[IBIS Ver]   5.1
[File name]   imx8mn_v1.ibs
[File Rev]   1.0
[Date]   Apr 12,2021
[Notes]   One-Section RLC
[Component] imx8mn_14x14_v1
[Manufacturer] Manufacturer_Name
[Package]
|   typ   min   max
R_pkg   0.39844   0.18702   0.658
L_pkg   2.971e-9   1.249e-9   5.232e-9
C_pkg   8.434e-13   5.175e-13   1.203e-12
[Pin]   Signal_name   model_name   R_pin   L_pin   C_pin
M19 NVCC_CLK POWER
K8 NVCC_DRAM POWER
K9 NVCC_DRAM POWER
L9 NVCC_DRAM POWER
M9 NVCC_DRAM POWER
N8 NVCC_DRAM POWER
N9 NVCC_DRAM POWER
P7 NVCC_DRAM POWER
R8 NVCC_DRAM POWER
R9 NVCC_DRAM POWER
T9 NVCC_DRAM POWER
U9 NVCC_DRAM POWER
V8 NVCC_DRAM POWER
V9 NVCC_DRAM POWER
H10 NVCC_ECSPI POWER
W22 NVCC_ENET POWER
W12 NVCC_GPIO1 POWER
J11 NVCC_I2C POWER
L19 NVCC_JTAG POWER
U19 NVCC_NAND POWER
V19 NVCC_SAI2 POWER
Y10 NVCC_SAI3 POWER
W17 NVCC_SAI5 POWER
V20 NVCC_SD1 POWER
V22 NVCC_SD2 POWER
J22 NVCC_SNVS_1P8 POWER
J12 NVCC_UART POWER
AB13 PVCC0_1P8 POWER
T19 PVCC1_1P8 POWER
J13 PVCC2_1P8 POWER
N19 VDD_24M_XTAL_1P8 POWER
AA14 VDD_ANA0_1P8 POWER
Y15 VDD_ANA0_1P8 POWER
N20 VDD_ANA1_1P8 POWER
P19 VDD_ANA1_1P8 POWER
L17 VDD_ANA_0P8 POWER
N17 VDD_ANA_0P8 POWER
R13 VDD_ARM POWER
R15 VDD_ARM POWER
T13 VDD_ARM POWER
T14 VDD_ARM POWER
T15 VDD_ARM POWER
U13 VDD_ARM POWER
U15 VDD_ARM POWER
V13 VDD_ARM POWER
V15 VDD_ARM POWER
V16 VDD_ARM POWER
W13 VDD_ARM POWER
W14 VDD_ARM POWER
W15 VDD_ARM POWER
W16 VDD_ARM POWER
P16 VDD_ARM_PLL_0P8 POWER
R19 VDD_ARM_PLL_1P8 POWER
J10 VDD_DRAM POWER
L10 VDD_DRAM POWER
N10 VDD_DRAM POWER
R10 VDD_DRAM POWER
U10 VDD_DRAM POWER
W10 VDD_DRAM POWER
P9 VDD_DRAM_PLL_0P8 POWER
P5 VDD_DRAM_PLL_1P8 POWER
P12 VDD_GPU POWER
R11 VDD_GPU POWER
U11 VDD_GPU POWER
V12 VDD_GPU POWER
W11 VDD_GPU POWER
J14 VDD_MIPI_0P8 POWER
J15 VDD_MIPI_1P2 POWER
H13 VDD_MIPI_1P8 POWER
K22 VDD_SNVS_0P8 POWER
K15 VDD_SOC POWER
K16 VDD_SOC POWER
L15 VDD_SOC POWER
L18 VDD_SOC POWER
M15 VDD_SOC POWER
N13 VDD_SOC POWER
N15 VDD_SOC POWER
N18 VDD_SOC POWER
R17 VDD_SOC POWER
R18 VDD_SOC POWER
U17 VDD_SOC POWER
U18 VDD_SOC POWER
J17 VDD_USB_0P8 POWER
H15 VDD_USB_1P8 POWER
K19 VDD_USB_3P3 POWER
P1 DRAM_VREF POWER
B27 24M_XTALI NC 0.51574 3.88E-09 9.69E-13
C26 24M_XTALO NC 0.47173 3.65E-09 9.10E-13
G26 BOOT_MODE0 PBIDIRHS_E33_33_NT_DR_H 0.46814 3.31E-09 8.70E-13
G27 BOOT_MODE1 PBIDIRHS_E33_33_NT_DR_H 0.42497 3.31E-09 8.83E-13
C27 BOOT_MODE2 PBIDIRHS_E33_33_NT_DR_H 0.658 4.64E-09 1.10E-12
D26 BOOT_MODE3 PBIDIRHS_E33_33_NT_DR_H 0.45096 3.50E-09 9.48E-13
H27 CLKIN1 PBIDIRHS_E33_33_NT_DR_H 0.42819 3.10E-09 8.46E-13
J27 CLKIN2 PBIDIRHS_E33_33_NT_DR_H 0.39512 2.88E-09 8.19E-13
H26 CLKOUT1 PBIDIRHS_E33_33_NT_DR_H 0.42258 3.09E-09 8.72E-13
J26 CLKOUT2 PBIDIRHS_E33_33_NT_DR_H 0.38896 2.86E-09 8.59E-13
F4 DRAM_AC00 CA_CK 0.48824 3.22E-09 9.34E-13
F5 DRAM_AC01 CA_CK 0.35707 2.39E-09 8.27E-13
K4 DRAM_AC02 CA_CK 0.39984 2.51E-09 6.33E-13
J4 DRAM_AC03 CA_CK 0.4301 2.77E-09 8.38E-13
L2 DRAM_AC04 CA_CK 0.36588 2.48E-09 7.90E-13
L1 DRAM_AC05 CA_CK 0.36576 2.54E-09 7.85E-13
F6 DRAM_AC06 CA_CK 0.4007 2.77E-09 8.84E-13
J5 DRAM_AC07 CA_CK 0.32797 2.10E-09 7.49E-13
J6 DRAM_AC08 CA_CK 0.37592 2.45E-09 7.51E-13
K6 DRAM_AC09 CA_CK 0.2687 1.75E-09 6.37E-13
E4 DRAM_AC10 CA_CK 0.47313 3.25E-09 1.07E-12
D5 DRAM_AC11 CA_CK 0.5424 3.66E-09 1.09E-12
N4 DRAM_AC12 CA_CK 0.31375 2.03E-09 7.30E-13
N5 DRAM_AC13 CA_CK 0.3154 2.11E-09 5.26E-13
K5 DRAM_AC14 CA_CK 0.38927 2.66E-09 8.12E-13
N6 DRAM_AC15 CA_CK 0.19955 1.25E-09 5.44E-13
M1 DRAM_AC16 CA_CK 0.35347 2.44E-09 7.55E-13
M2 DRAM_AC17 CA_CK 0.358 2.43E-09 7.51E-13
N2 DRAM_AC19 CA_CK 0.40801 2.75E-09 7.90E-13
AB4 DRAM_AC20 CA_CK 0.42345 3.02E-09 1.01E-12
AB5 DRAM_AC21 CA_CK 0.42752 3.07E-09 9.99E-13
W4 DRAM_AC22 CA_CK 0.4158 2.93E-09 8.70E-13
V4 DRAM_AC23 CA_CK 0.32528 2.28E-09 8.23E-13
U2 DRAM_AC24 CA_CK 0.39035 2.60E-09 7.87E-13
U1 DRAM_AC25 CA_CK 0.38541 2.61E-09 8.04E-13
N1 DRAM_AC26 CA_CK 0.44985 3.23E-09 9.76E-13
R6 DRAM_AC27 CA_CK 0.25296 1.74E-09 5.79E-13
W6 DRAM_AC28 CA_CK 0.24654 1.73E-09 6.92E-13
V6 DRAM_AC29 CA_CK 0.2963 2.07E-09 6.79E-13
AC4 DRAM_AC30 CA_CK 0.49352 3.59E-09 1.07E-12
AD5 DRAM_AC31 CA_CK 0.4395 3.25E-09 1.10E-12
R4 DRAM_AC32 CA_CK 0.27402 1.95E-09 7.28E-13
R5 DRAM_AC33 CA_CK 0.33648 2.47E-09 7.04E-13
T1 DRAM_AC34 CA_CK 0.33909 2.47E-09 8.79E-13
T2 DRAM_AC35 CA_CK 0.4206 3.03E-09 9.57E-13
V5 DRAM_AC36 CA_CK 0.21143 1.53E-09 5.18E-13
W5 DRAM_AC37 CA_CK 0.27343 2.01E-09 7.34E-13
AB6 DRAM_AC38 CA_CK 0.3378 2.47E-09 7.95E-13
R2 DRAM_ALERT_N CA_CK 0.32975 2.21E-09 7.44E-13
A4 DRAM_DM0 DQ_DQS 0.49985 3.46E-09 1.04E-12
F1 DRAM_DM1 DQ_DQS 0.5397 3.63E-09 1.05E-12
A5 DRAM_DQ00 DQ_DQS 0.39147 2.99E-09 8.20E-13
B5 DRAM_DQ01 DQ_DQS 0.3615 2.50E-09 8.23E-13
D2 DRAM_DQ02 DQ_DQS 0.47251 3.12E-09 9.96E-13
D1 DRAM_DQ03 DQ_DQS 0.41907 2.95E-09 9.98E-13
C1 DRAM_DQ04 DQ_DQS 0.59741 3.79E-09 1.09E-12
B1 DRAM_DQ05 DQ_DQS 0.54423 3.70E-09 9.92E-13
A3 DRAM_DQ06 DQ_DQS 0.59637 3.94E-09 1.17E-12
B4 DRAM_DQ07 DQ_DQS 0.44773 2.99E-09 1.01E-12
F2 DRAM_DQ08 DQ_DQS 0.41874 2.65E-09 8.49E-13
G2 DRAM_DQ09 DQ_DQS 0.49278 3.11E-09 8.75E-13
J1 DRAM_DQ10 DQ_DQS 0.40348 2.71E-09 9.07E-13
J2 DRAM_DQ11 DQ_DQS 0.46658 2.91E-09 8.48E-13
K2 DRAM_DQ12 DQ_DQS 0.37348 2.33E-09 7.90E-13
K1 DRAM_DQ13 DQ_DQS 0.47478 3.06E-09 8.57E-13
E1 DRAM_DQ14 DQ_DQS 0.48488 3.33E-09 1.12E-12
E2 DRAM_DQ15 DQ_DQS 0.45234 3.01E-09 1.02E-12
B2 DRAM_DQS0_N DQ_DQS 0.53019 3.56E-09 1.07E-12
A2 DRAM_DQS0_P DQ_DQS 0.53145 3.58E-09 1.06E-12
H1 DRAM_DQS1_N DQ_DQS 0.40944 3.10E-09 8.31E-13
G1 DRAM_DQS1_P DQ_DQS 0.40431 3.20E-09 8.34E-13
R1 DRAM_RESET_N CA_CK 0.3454 2.35E-09 7.49E-13
P2 DRAM_ZN CA_CK 0.23974 1.79E-09 7.30E-13
A7 ECSPI1_MISO PBIDIRHS_E33_33_NT_DR_V 0.37355 2.89E-09 7.69E-13
B7 ECSPI1_MOSI PBIDIRHS_E33_33_NT_DR_V 0.33402 2.36E-09 7.74E-13
D6 ECSPI1_SCLK PBIDIRHS_E33_33_NT_DR_V 0.29824 2.14E-09 8.07E-13
B6 ECSPI1_SS0 PBIDIRHS_E33_33_NT_DR_V 0.33367 2.42E-09 8.63E-13
A8 ECSPI2_MISO PBIDIRHS_E33_33_NT_DR_V 0.351 2.53E-09 8.75E-13
B8 ECSPI2_MOSI PBIDIRHS_E33_33_NT_DR_V 0.34979 2.52E-09 8.27E-13
E6 ECSPI2_SCLK PBIDIRHS_E33_33_NT_DR_V 0.24339 1.77E-09 7.01E-13
A6 ECSPI2_SS0 PBIDIRHS_E33_33_NT_DR_V 0.378 2.72E-09 9.37E-13
AC27 ENET_MDC PBIDIRHS_E33_33_NT_DR_V 0.49185 3.73E-09 1.02E-12
AB27 ENET_MDIO PBIDIRHS_E33_33_NT_DR_V 0.52367 3.84E-09 1.03E-12
AE27 ENET_RD0 PBIDIRHS_E33_33_NT_DR_V 0.60251 4.83E-09 1.15E-12
AD27 ENET_RD1 PBIDIRHS_E33_33_NT_DR_V 0.58514 4.47E-09 1.11E-12
AD26 ENET_RD2 PBIDIRHS_E33_33_NT_DR_V 0.54339 4.25E-09 1.02E-12
AC26 ENET_RD3 PBIDIRHS_E33_33_NT_DR_V 0.50617 4.39E-09 9.34E-13
AE26 ENET_RXC PBIDIRHS_E33_33_NT_DR_V 0.58821 4.99E-09 1.00E-12
AF27 ENET_RX_CTL PBIDIRHS_E33_33_NT_DR_V 0.6411 4.81E-09 1.17E-12
AG26 ENET_TD0 PBIDIRHS_E33_33_NT_DR_V 0.63183 5.23E-09 1.20E-12
AF26 ENET_TD1 PBIDIRHS_E33_33_NT_DR_V 0.53971 4.66E-09 1.03E-12
AG25 ENET_TD2 PBIDIRHS_E33_33_NT_DR_V 0.56983 5.01E-09 1.01E-12
AF25 ENET_TD3 PBIDIRHS_E33_33_NT_DR_V 0.53389 4.38E-09 1.04E-12
AG24 ENET_TXC PBIDIRHS_E33_33_NT_DR_V 0.60522 4.99E-09 1.09E-12
AF24 ENET_TX_CTL PBIDIRHS_E33_33_NT_DR_V 0.49602 3.94E-09 9.36E-13
AG14 GPIO1_IO00 PBIDIRHS_E33_33_NT_DR_V 0.47303 3.55E-09 1.03E-12
AF14 GPIO1_IO01 PBIDIRHS_E33_33_NT_DR_V 0.49773 3.62E-09 9.72E-13
AG13 GPIO1_IO02 PBIDIRHS_E33_33_NT_DR_V 0.42117 3.18E-09 9.11E-13
AF13 GPIO1_IO03 PBIDIRHS_E33_33_NT_DR_V 0.43028 3.16E-09 8.20E-13
AG12 GPIO1_IO04 PBIDIRHS_E33_33_NT_DR_V 0.44738 3.29E-09 9.53E-13
AF12 GPIO1_IO05 PBIDIRHS_E33_33_NT_DR_V 0.42301 3.03E-09 8.41E-13
AG11 GPIO1_IO06 PBIDIRHS_E33_33_NT_DR_V 0.38341 2.96E-09 7.42E-13
AF11 GPIO1_IO07 PBIDIRHS_E33_33_NT_DR_V 0.42212 3.04E-09 7.78E-13
AG10 GPIO1_IO08 PBIDIRHS_E33_33_NT_DR_V 0.42061 3.41E-09 7.40E-13
AF10 GPIO1_IO09 PBIDIRHS_E33_33_NT_DR_V 0.48934 3.59E-09 9.08E-13
AD10 GPIO1_IO10 PBIDIRHS_E33_33_NT_DR_V 0.32648 2.56E-09 7.47E-13
AC10 GPIO1_IO11 PBIDIRHS_E33_33_NT_DR_V 0.40226 3.02E-09 8.33E-13
AB10 GPIO1_IO12 PBIDIRHS_E33_33_NT_DR_V 0.29622 2.30E-09 6.74E-13
AD9 GPIO1_IO13 PBIDIRHS_E33_33_NT_DR_V 0.40673 3.04E-09 8.24E-13
AC9 GPIO1_IO14 PBIDIRHS_E33_33_NT_DR_V 0.34159 2.68E-09 7.60E-13
AB9 GPIO1_IO15 PBIDIRHS_E33_33_NT_DR_V 0.38348 2.87E-09 7.64E-13
E9 I2C1_SCL PBIDIRHS_E33_33_NT_DR_V 0.25158 2.14E-09 6.92E-13
F9 I2C1_SDA PBIDIRHS_E33_33_NT_DR_V 0.19616 1.61E-09 6.06E-13
D10 I2C2_SCL PBIDIRHS_E33_33_NT_DR_V 0.27825 2.30E-09 7.25E-13
D9 I2C2_SDA PBIDIRHS_E33_33_NT_DR_V 0.27493 2.22E-09 7.43E-13
E10 I2C3_SCL PBIDIRHS_E33_33_NT_DR_V 0.21555 1.65E-09 5.84E-13
F10 I2C3_SDA PBIDIRHS_E33_33_NT_DR_V 0.19827 1.70E-09 5.71E-13
D13 I2C4_SCL PBIDIRHS_E33_33_NT_DR_V 0.33107 2.61E-09 8.61E-13
E13 I2C4_SDA PBIDIRHS_E33_33_NT_DR_V 0.29585 2.52E-09 7.61E-13
D27 JTAG_MOD PBIDIRHS_E33_33_NT_DR_V 0.60254 4.45E-09 1.11E-12
F26 JTAG_TCK PBIDIRHS_E33_33_NT_DR_V 0.4046 3.09E-09 8.46E-13
E27 JTAG_TDI PBIDIRHS_E33_33_NT_DR_V 0.50933 3.80E-09 9.77E-13
E26 JTAG_TDO PBIDIRHS_E33_33_NT_DR_V 0.55324 4.11E-09 1.02E-12
F27 JTAG_TMS PBIDIRHS_E33_33_NT_DR_V 0.52515 3.82E-09 9.81E-13
A16 MIPI_CSI_CLK_N DPHY_RX 0.45964 3.21E-09 8.86E-13
B16 MIPI_CSI_CLK_P DPHY_RX 0.44956 3.14E-09 8.89E-13
A14 MIPI_CSI_D0_N DPHY_RX 0.44549 3.14E-09 8.76E-13
B14 MIPI_CSI_D0_P DPHY_RX 0.4516 3.13E-09 8.63E-13
A15 MIPI_CSI_D1_N DPHY_RX 0.45153 3.18E-09 8.87E-13
B15 MIPI_CSI_D1_P DPHY_RX 0.46295 3.20E-09 8.68E-13
A17 MIPI_CSI_D2_N DPHY_RX 0.4619 3.26E-09 8.75E-13
B17 MIPI_CSI_D2_P DPHY_RX 0.45927 3.18E-09 8.77E-13
A18 MIPI_CSI_D3_N DPHY_RX 0.45552 3.23E-09 8.74E-13
B18 MIPI_CSI_D3_P DPHY_RX 0.45125 3.18E-09 8.80E-13
A11 MIPI_DSI_CLK_N DPHY_TX 0.4522 3.02E-09 8.88E-13
B11 MIPI_DSI_CLK_P DPHY_TX 0.44443 2.98E-09 8.65E-13
A9 MIPI_DSI_D0_N DPHY_TX 0.44051 3.11E-09 8.90E-13
B9 MIPI_DSI_D0_P DPHY_TX 0.4461 3.17E-09 8.59E-13
A10 MIPI_DSI_D1_N DPHY_TX 0.44518 3.03E-09 8.77E-13
B10 MIPI_DSI_D1_P DPHY_TX 0.44943 3.06E-09 8.56E-13
A12 MIPI_DSI_D2_N DPHY_TX 0.45489 3.23E-09 8.88E-13
B12 MIPI_DSI_D2_P DPHY_TX 0.46388 3.01E-09 8.79E-13
A13 MIPI_DSI_D3_N DPHY_TX 0.44597 3.26E-09 8.85E-13
B13 MIPI_DSI_D3_P DPHY_TX 0.45687 3.24E-09 8.67E-13
D15 MIPI_VREG_CAP NC 0.33053 2.45E-09 7.14E-13
N22 NAND_ALE PBIDIRHS_E33_33_NT_DR_H 0.26209 1.92E-09 5.56E-13
N24 NAND_CE0_B PBIDIRHS_E33_33_NT_DR_H 0.3626 3.19E-09 7.69E-13
P27 NAND_CE1_B PBIDIRHS_E33_33_NT_DR_H 0.41324 3.16E-09 8.06E-13
M27 NAND_CE2_B PBIDIRHS_E33_33_NT_DR_H 0.50235 3.88E-09 8.77E-13
L27 NAND_CE3_B PBIDIRHS_E33_33_NT_DR_H 0.41619 3.33E-09 9.27E-13
K27 NAND_CLE PBIDIRHS_E33_33_NT_DR_H 0.44944 3.60E-09 9.50E-13
P23 NAND_DATA00 PBIDIRHS_E33_33_NT_DR_H 0.23195 2.34E-09 6.09E-13
K24 NAND_DATA01 PBIDIRHS_E33_33_NT_DR_H 0.30636 2.35E-09 7.32E-13
K23 NAND_DATA02 PBIDIRHS_E33_33_NT_DR_H 0.32853 2.76E-09 8.04E-13
N23 NAND_DATA03 PBIDIRHS_E33_33_NT_DR_H 0.22735 1.98E-09 5.70E-13
M26 NAND_DATA04 PBIDIRHS_E33_33_NT_DR_H 0.43592 3.78E-09 8.40E-13
L26 NAND_DATA05 PBIDIRHS_E33_33_NT_DR_H 0.40519 3.05E-09 8.29E-13
K26 NAND_DATA06 PBIDIRHS_E33_33_NT_DR_H 0.41314 3.66E-09 9.50E-13
N26 NAND_DATA07 PBIDIRHS_E33_33_NT_DR_H 0.41424 3.08E-09 8.08E-13
R22 NAND_DQS PBIDIRHS_E33_33_NT_DR_H 0.28012 2.14E-09 6.66E-13
P26 NAND_READY_B PBIDIRHS_E33_33_NT_DR_H 0.31826 2.47E-09 7.40E-13
N27 NAND_RE_B PBIDIRHS_E33_33_NT_DR_H 0.44902 3.43E-09 8.46E-13
R26 NAND_WE_B PBIDIRHS_E33_33_NT_DR_H 0.49038 3.54E-09 9.33E-13
R27 NAND_WP_B PBIDIRHS_E33_33_NT_DR_H 0.3616 2.86E-09 8.09E-13
A25 ONOFF PINC_E33_33_NT_DR_H 0.42391 3.27E-09 9.04E-13
A24 PMIC_ON_REQ PBIDIR_E33_33_NT_DR_H 0.42415 3.44E-09 7.76E-13
E24 PMIC_STBY_REQ PBIDIR_E33_33_NT_DR_H 0.43218 3.22E-09 8.78E-13
B24 POR_B PINC_E33_33_NT_DR_H 0.43987 3.79E-09 9.00E-13
F24 RTC_RESET_B PINC_E33_33_NT_DR_H 0.29095 2.49E-09 7.04E-13
A26 RTC_XTALI NC 0.50843 4.03E-09 9.60E-13
B25 RTC_XTALO NC 0.48113 3.81E-09 9.71E-13
AD19 SAI2_MCLK PBIDIRHS_E33_33_NT_DR_V 0.34257 2.69E-09 7.35E-13
AB22 SAI2_RXC PBIDIRHS_E33_33_NT_DR_V 0.47663 3.51E-09 8.91E-13
AC24 SAI2_RXD0 PBIDIRHS_E33_33_NT_DR_V 0.56459 4.37E-09 1.02E-12
AC19 SAI2_RXFS PBIDIRHS_E33_33_NT_DR_V 0.30707 2.36E-09 6.89E-13
AD22 SAI2_TXC PBIDIRHS_E33_33_NT_DR_V 0.46249 3.50E-09 9.07E-13
AC22 SAI2_TXD0 PBIDIRHS_E33_33_NT_DR_V 0.48787 3.55E-09 9.44E-13
AD23 SAI2_TXFS PBIDIRHS_E33_33_NT_DR_V 0.56772 4.24E-09 1.04E-12
AD6 SAI3_MCLK PBIDIRHS_E33_33_NT_DR_V 0.33969 2.39E-09 7.88E-13
AG7 SAI3_RXC PBIDIRHS_E33_33_NT_DR_V 0.37044 2.73E-09 8.81E-13
AF7 SAI3_RXD PBIDIRHS_E33_33_NT_DR_V 0.36591 2.65E-09 8.38E-13
AG8 SAI3_RXFS PBIDIRHS_E33_33_NT_DR_V 0.36577 2.56E-09 8.68E-13
AG6 SAI3_TXC PBIDIRHS_E33_33_NT_DR_V 0.39305 2.73E-09 9.47E-13
AF6 SAI3_TXD PBIDIRHS_E33_33_NT_DR_V 0.35362 2.42E-09 8.58E-13
AC6 SAI3_TXFS PBIDIRHS_E33_33_NT_DR_V 0.34927 2.54E-09 8.07E-13
AD15 SAI5_MCLK PBIDIRHS_E33_33_NT_DR_V 0.29891 2.34E-09 7.29E-13
AC15 SAI5_RXC PBIDIRHS_E33_33_NT_DR_V 0.32942 2.52E-09 6.46E-13
AD18 SAI5_RXD0 PBIDIRHS_E33_33_NT_DR_V 0.33327 2.69E-09 7.85E-13
AC14 SAI5_RXD1 PBIDIRHS_E33_33_NT_DR_V 0.31434 2.41E-09 5.75E-13
AD13 SAI5_RXD2 PBIDIRHS_E33_33_NT_DR_V 0.27461 2.16E-09 6.41E-13
AC13 SAI5_RXD3 PBIDIRHS_E33_33_NT_DR_V 0.29893 2.29E-09 6.19E-13
AB15 SAI5_RXFS PBIDIRHS_E33_33_NT_DR_V 0.2232 1.92E-09 5.41E-13
V26 SD1_CLK PBIDIRHS_E33_33_NT_DR_V 0.25323 2.53E-09 6.55E-13
V27 SD1_CMD PBIDIRHS_E33_33_NT_DR_V 0.33989 3.17E-09 6.87E-13
Y27 SD1_DATA0 PBIDIRHS_E33_33_NT_DR_V 0.4466 3.67E-09 9.99E-13
Y26 SD1_DATA1 PBIDIRHS_E33_33_NT_DR_V 0.46127 3.88E-09 9.96E-13
T27 SD1_DATA2 PBIDIRHS_E33_33_NT_DR_V 0.29453 2.22E-09 7.43E-13
T26 SD1_DATA3 PBIDIRHS_E33_33_NT_DR_V 0.27353 2.09E-09 6.88E-13
U27 SD1_DATA4 PBIDIRHS_E33_33_NT_DR_V 0.28781 2.72E-09 7.19E-13
U26 SD1_DATA5 PBIDIRHS_E33_33_NT_DR_V 0.33696 3.14E-09 7.50E-13
W27 SD1_DATA6 PBIDIRHS_E33_33_NT_DR_V 0.38309 3.50E-09 8.88E-13
W26 SD1_DATA7 PBIDIRHS_E33_33_NT_DR_V 0.35732 3.22E-09 8.21E-13
R23 SD1_RESET_B PBIDIRHS_E33_33_NT_DR_V 0.23123 2.31E-09 6.06E-13
R24 SD1_STROBE PBIDIRHS_E33_33_NT_DR_V 0.28213 2.64E-09 6.81E-13
AA26 SD2_CD_B PBIDIRHS_E33_33_NT_DR_V 0.44753 3.49E-09 8.75E-13
W23 SD2_CLK PBIDIRHS_E33_33_NT_DR_V 0.29617 2.07E-09 6.75E-13
W24 SD2_CMD PBIDIRHS_E33_33_NT_DR_V 0.45316 3.15E-09 8.91E-13
AB23 SD2_DATA0 PBIDIRHS_E33_33_NT_DR_V 0.35157 2.55E-09 7.17E-13
AB24 SD2_DATA1 PBIDIRHS_E33_33_NT_DR_V 0.45317 3.12E-09 8.55E-13
V24 SD2_DATA2 PBIDIRHS_E33_33_NT_DR_V 0.37973 2.67E-09 8.35E-13
V23 SD2_DATA3 PBIDIRHS_E33_33_NT_DR_V 0.39303 2.73E-09 8.15E-13
AB26 SD2_RESET_B PBIDIRHS_E33_33_NT_DR_V 0.43121 3.09E-09 9.09E-13
AA27 SD2_WP PBIDIRHS_E33_33_NT_DR_V 0.3967 3.26E-09 8.41E-13
AF8 SPDIF_EXT_CLK PBIDIRHS_E33_33_NT_DR_V 0.33644 2.30E-09 7.70E-13
AG9 SPDIF_RX PBIDIRHS_E33_33_NT_DR_V 0.37793 2.84E-09 8.39E-13
AF9 SPDIF_TX PBIDIRHS_E33_33_NT_DR_V 0.33891 2.55E-09 7.08E-13
J24 TSENSOR_RES_EXT NC 0.38573 3.32E-09 7.36E-13
J23 TSENSOR_TEST_OUT NC 0.30696 2.91E-09 6.90E-13
E14 UART1_RXD PBIDIRHS_E33_33_NT_DR_V 0.2878 2.84E-09 7.19E-13
F13 UART1_TXD PBIDIRHS_E33_33_NT_DR_V 0.18702 1.72E-09 5.69E-13
F15 UART2_RXD PBIDIRHS_E33_33_NT_DR_V 0.2143 2.05E-09 6.16E-13
E15 UART2_TXD PBIDIRHS_E33_33_NT_DR_V 0.32045 2.80E-09 8.26E-13
E18 UART3_RXD PBIDIRHS_E33_33_NT_DR_V 0.35564 3.09E-09 8.91E-13
D18 UART3_TXD PBIDIRHS_E33_33_NT_DR_V 0.43732 3.72E-09 1.04E-12
F19 UART4_RXD PBIDIRHS_E33_33_NT_DR_V 0.30696 2.29E-09 8.00E-13
F18 UART4_TXD PBIDIRHS_E33_33_NT_DR_V 0.35022 3.04E-09 8.61E-13
A22 USB1_DN USB2_HS_IBIS 0.39952 2.69E-09 8.72E-13
B22 USB1_DP USB2_HS_IBIS 0.41181 2.68E-09 8.58E-13
D22 USB1_ID NC 0.31957 2.36E-09 7.60E-13
E19 USB1_TXRTUNE NC 0.31315 2.30E-09 8.37E-13
F22 USB1_VBUS NC 0.25661 2.00E-09 6.88E-13
A1 VSS GND
A27 VSS GND
AA7 VSS GND
AA9 VSS GND
AA10 VSS GND
AA13 VSS GND
AA15 VSS GND
AA18 VSS GND
AA19 VSS GND
AA21 VSS GND
AB3 VSS GND
AB25 VSS GND
AC3 VSS GND
AC25 VSS GND
AE2 VSS GND
AE5 VSS GND
AE6 VSS GND
AE9 VSS GND
AE10 VSS GND
AE13 VSS GND
AE14 VSS GND
AE15 VSS GND
AE18 VSS GND
AE19 VSS GND
AE22 VSS GND
AE23 VSS GND
AF3 VSS GND
AG1 VSS GND
AG27 VSS GND
B3 VSS GND
B26 VSS GND
C2 VSS GND
C5 VSS GND
C6 VSS GND
C9 VSS GND
C10 VSS GND
C13 VSS GND
C14 VSS GND
C15 VSS GND
C18 VSS GND
C19 VSS GND
C22 VSS GND
C23 VSS GND
E3 VSS GND
E25 VSS GND
F3 VSS GND
F25 VSS GND
G7 VSS GND
G9 VSS GND
G10 VSS GND
G13 VSS GND
G15 VSS GND
G18 VSS GND
G19 VSS GND
G21 VSS GND
H2 VSS GND
H18 VSS GND
J3 VSS GND
J7 VSS GND
J21 VSS GND
J25 VSS GND
K3 VSS GND
K7 VSS GND
K20 VSS GND
K21 VSS GND
K25 VSS GND
L12 VSS GND
L16 VSS GND
M12 VSS GND
M16 VSS GND
N3 VSS GND
N7 VSS GND
N12 VSS GND
N16 VSS GND
N21 VSS GND
N25 VSS GND
P3 VSS GND
P13 VSS GND
P15 VSS GND
P21 VSS GND
P25 VSS GND
R3 VSS GND
R7 VSS GND
R12 VSS GND
R16 VSS GND
R20 VSS GND
R21 VSS GND
R25 VSS GND
T12 VSS GND
T16 VSS GND
U12 VSS GND
U16 VSS GND
V3 VSS GND
V7 VSS GND
V21 VSS GND
V25 VSS GND
W3 VSS GND
W7 VSS GND
W21 VSS GND
W25 VSS GND
Y2 VSS GND
Y13 VSS GND
Y18 VSS GND
[Diff_pin] inv_pin vdiff tdelay_typ tdelay_min tdelay_max
L2 L1 0.140V 0ns NA NA
M1 M2 0.140V 0ns NA NA
AB4 AB5 0.140V 0ns NA NA
U2 U1 0.140V 0ns NA NA
A2 B2 0.140V 0ns NA NA
G1 H1 0.140V 0ns NA NA
B16 A16 NA NA NA NA
B14 A14 NA NA NA NA
B15 A15 NA NA NA NA
B17 A17 NA NA NA NA
B18 A18 NA NA NA NA
B11 A11 NA NA NA NA
B9 A9 NA NA NA NA
B10 A10 NA NA NA NA
B12 A12 NA NA NA NA
B13 A13 NA NA NA NA
B22 A22 150.000mV 0ns NA NA
|END COMPONENT
[Component] imx8mn_11x11_v1
[Manufacturer] Manufacturer_Name
[Package]
|   typ   min   max
R_pkg   0.25043   0.042363   0.44547
L_pkg   1.837e-9   3.367e-10   3.156e-9
C_pkg   5.291e-13   2.309e-13   8.779e-13
[Pin]   Signal_name   model_name   R_pin   L_pin   C_pin
L15 NVCC_CLK_JTAG_PVCC_1P8 POWER
G6 NVCC_DRAM POWER
J6 NVCC_DRAM POWER
J7 NVCC_DRAM POWER
L6 NVCC_DRAM POWER
N6 NVCC_DRAM POWER
N7 NVCC_DRAM POWER
R6 NVCC_DRAM POWER
G8 NVCC_ECSPI POWER
R12 NVCC_ENET_GPIO_SAI2 POWER
G10 NVCC_I2C_UART POWER
R10 NVCC_SAI3_SAI5 POWER
N15 NVCC_SD1_NAND POWER
R16 NVCC_SD2 POWER
G14 NVCC_SNVS_1P8 POWER
R14 VDD_ANA0_ARM_PLL_1P8 POWER
G12 VDD_ANA1_XTAL_MIPI_USB_1P8 POWER
L7 VDD_DRAM_PLL_1P8 POWER
F12 VDD_MIPI_1P2 POWER
J15 VDD_SNVS_0P8 POWER
J9 VDD_SOC POWER
J10 VDD_SOC POWER
J11 VDD_SOC POWER
J12 VDD_SOC POWER
J13 VDD_SOC POWER
K10 VDD_SOC POWER
K12 VDD_SOC POWER
L9 VDD_SOC POWER
L10 VDD_SOC POWER
L12 VDD_SOC POWER
L13 VDD_SOC POWER
M10 VDD_SOC POWER
M12 VDD_SOC POWER
N9 VDD_SOC POWER
N10 VDD_SOC POWER
N11 VDD_SOC POWER
N12 VDD_SOC POWER
N13 VDD_SOC POWER
F14 VDD_USB_3P3 POWER
B21 24M_XTALI NC 0.34402 2.37E-09 6.75E-13
C20 24M_XTALO NC 0.31968 2.15E-09 6.17E-13
G16 BOOT_MODE0 PBIDIRHS_E33_33_NT_DR_H 0.31347 2.14E-09 6.06E-13
G18 BOOT_MODE1 PBIDIRHS_E33_33_NT_DR_H 0.18609 1.14E-09 3.66E-13
F16 BOOT_MODE2 PBIDIRHS_E33_33_NT_DR_H 0.28476 2.00E-09 5.96E-13
G17 BOOT_MODE3 PBIDIRHS_E33_33_NT_DR_H 0.17659 1.11E-09 3.76E-13
E20 CLKIN1 PBIDIRHS_E33_33_NT_DR_H 0.27193 1.96E-09 6.00E-13
F20 CLKIN2 PBIDIRHS_E33_33_NT_DR_H 0.25609 1.82E-09 5.63E-13
E21 CLKOUT1 PBIDIRHS_E33_33_NT_DR_H 0.33318 2.45E-09 6.56E-13
F21 CLKOUT2 PBIDIRHS_E33_33_NT_DR_H 0.2846 2.07E-09 5.82E-13
P1 DRAM_AC00 CA_CK 0.40386 2.77E-09 7.66E-13
N1 DRAM_AC01 CA_CK 0.28071 1.99E-09 6.28E-13
N2 DRAM_AC02 CA_CK 0.36629 2.49E-09 6.72E-13
P2 DRAM_AC03 CA_CK 0.37274 2.44E-09 7.14E-13
G5 DRAM_AC04 CA_CK 0.23444 1.60E-09 5.56E-13
G4 DRAM_AC05 CA_CK 0.24211 1.59E-09 5.38E-13
D4 DRAM_AC06 CA_CK 0.4048 2.79E-09 8.78E-13
E4 DRAM_AC07 CA_CK 0.29365 2.12E-09 7.32E-13
R1 DRAM_AC08 CA_CK 0.37065 2.45E-09 7.38E-13
R2 DRAM_AC09 CA_CK 0.28467 2.06E-09 6.90E-13
M2 DRAM_AC10 CA_CK 0.20747 1.42E-09 4.72E-13
L2 DRAM_AC11 CA_CK 0.25757 1.60E-09 5.37E-13
L1 DRAM_AC12 CA_CK 0.22609 1.59E-09 5.57E-13
M1 DRAM_AC13 CA_CK 0.28995 1.86E-09 5.60E-13
Y1 DRAM_AC14 CA_CK 0.44547 3.09E-09 8.72E-13
L5 DRAM_AC15 CA_CK 0.098799 5.93E-10 3.04E-13
J4 DRAM_AC16 CA_CK 0.12494 8.94E-10 3.89E-13
J5 DRAM_AC17 CA_CK 0.121 8.55E-10 3.89E-13
T1 DRAM_AC20 CA_CK 0.26122 1.77E-09 5.42E-13
T2 DRAM_AC21 CA_CK 0.26548 1.75E-09 5.37E-13
R4 DRAM_AC23 CA_CK 0.15935 1.03E-09 4.12E-13
Y2 DRAM_AC24 CA_CK 0.4216 2.81E-09 7.67E-13
AA2 DRAM_AC25 CA_CK 0.41593 2.81E-09 7.58E-13
W2 DRAM_AC26 CA_CK 0.39256 2.67E-09 7.74E-13
AA3 DRAM_AC28 CA_CK 0.35735 2.50E-09 6.80E-13
V4 DRAM_AC29 CA_CK 0.32096 1.98E-09 5.72E-13
W1 DRAM_AC30 CA_CK 0.38896 2.55E-09 7.09E-13
Y3 DRAM_AC31 CA_CK 0.27853 1.95E-09 6.01E-13
R5 DRAM_AC32 CA_CK 0.11867 7.05E-10 3.21E-13
U2 DRAM_AC33 CA_CK 0.30937 1.98E-09 6.19E-13
V2 DRAM_AC34 CA_CK 0.24755 1.73E-09 6.17E-13
U4 DRAM_AC35 CA_CK 0.25036 1.51E-09 5.12E-13
V1 DRAM_AC36 CA_CK 0.25904 1.93E-09 6.62E-13
N5 DRAM_ALERT_N CA_CK 0.14686 9.37E-10 3.79E-13
B2 DRAM_DM0 DQ_DQS 0.35964 2.27E-09 6.61E-13
H2 DRAM_DM1 DQ_DQS 0.26478 1.70E-09 5.13E-13
B3 DRAM_DQ00 DQ_DQS 0.25328 1.76E-09 5.19E-13
A2 DRAM_DQ01 DQ_DQS 0.29373 2.02E-09 6.20E-13
A3 DRAM_DQ02 DQ_DQS 0.38242 2.44E-09 6.61E-13
B4 DRAM_DQ03 DQ_DQS 0.27322 1.76E-09 5.74E-13
E2 DRAM_DQ04 DQ_DQS 0.36067 2.27E-09 6.55E-13
D1 DRAM_DQ05 DQ_DQS 0.29299 1.91E-09 6.01E-13
C1 DRAM_DQ06 DQ_DQS 0.39163 2.47E-09 6.69E-13
D2 DRAM_DQ07 DQ_DQS 0.25229 1.67E-09 5.00E-13
G1 DRAM_DQ08 DQ_DQS 0.29319 2.01E-09 5.56E-13
H1 DRAM_DQ09 DQ_DQS 0.37061 2.38E-09 6.50E-13
J1 DRAM_DQ10 DQ_DQS 0.27276 1.85E-09 6.05E-13
J2 DRAM_DQ11 DQ_DQS 0.29602 1.77E-09 5.42E-13
K1 DRAM_DQ12 DQ_DQS 0.23332 1.68E-09 5.28E-13
K2 DRAM_DQ13 DQ_DQS 0.27712 1.97E-09 5.89E-13
F2 DRAM_DQ14 DQ_DQS 0.27937 2.05E-09 6.54E-13
E1 DRAM_DQ15 DQ_DQS 0.31045 2.27E-09 6.51E-13
C2 DRAM_DQS0_N DQ_DQS 0.339 2.24E-09 6.54E-13
B1 DRAM_DQS0_P DQ_DQS 0.34234 2.22E-09 6.33E-13
F1 DRAM_DQS1_N DQ_DQS 0.28234 1.89E-09 5.74E-13
G2 DRAM_DQS1_P DQ_DQS 0.28233 1.92E-09 5.59E-13
N4 DRAM_RESET_N CA_CK 0.14028 9.16E-10 3.91E-13
L4 DRAM_VREF NC 0.10007 7.90E-10 4.11E-13
U1 DRAM_ZN CA_CK 0.23566 1.94E-09 6.71E-13
D6 ECSPI1_MISO PBIDIRHS_E33_33_NT_DR_V 0.1392 1.29E-09 4.61E-13
F6 ECSPI1_MOSI PBIDIRHS_E33_33_NT_DR_V 0.056326 4.41E-10 3.14E-13
E6 ECSPI1_SCLK PBIDIRHS_E33_33_NT_DR_V 0.10924 9.88E-10 3.97E-13
B6 ECSPI1_SS0 PBIDIRHS_E33_33_NT_DR_V 0.15797 1.50E-09 4.96E-13
B5 ECSPI2_MISO PBIDIRHS_E33_33_NT_DR_V 0.16655 1.32E-09 5.21E-13
A6 ECSPI2_MOSI PBIDIRHS_E33_33_NT_DR_V 0.19777 1.83E-09 5.40E-13
A4 ECSPI2_SCLK PBIDIRHS_E33_33_NT_DR_V 0.20686 1.66E-09 5.79E-13
A5 ECSPI2_SS0 PBIDIRHS_E33_33_NT_DR_V 0.21084 1.90E-09 5.71E-13
Y18 ENET_MDC PBIDIRHS_E33_33_NT_DR_V 0.27153 2.24E-09 5.55E-13
T16 ENET_MDIO PBIDIRHS_E33_33_NT_DR_V 0.22013 1.69E-09 4.14E-13
AA19 ENET_RD0 PBIDIRHS_E33_33_NT_DR_V 0.4001 3.16E-09 7.28E-13
Y15 ENET_RD1 PBIDIRHS_E33_33_NT_DR_V 0.25196 2.05E-09 5.43E-13
Y16 ENET_RD2 PBIDIRHS_E33_33_NT_DR_V 0.25138 2.06E-09 5.43E-13
AA16 ENET_RD3 PBIDIRHS_E33_33_NT_DR_V 0.28001 2.36E-09 5.90E-13
U16 ENET_RXC PBIDIRHS_E33_33_NT_DR_V 0.30232 2.35E-09 5.81E-13
V16 ENET_RX_CTL PBIDIRHS_E33_33_NT_DR_V 0.31447 2.41E-09 5.92E-13
U18 ENET_TD0 PBIDIRHS_E33_33_NT_DR_V 0.30147 2.33E-09 5.36E-13
AA18 ENET_TD1 PBIDIRHS_E33_33_NT_DR_V 0.29618 2.48E-09 6.03E-13
V18 ENET_TD2 PBIDIRHS_E33_33_NT_DR_V 0.31084 2.44E-09 5.86E-13
AA17 ENET_TD3 PBIDIRHS_E33_33_NT_DR_V 0.28116 2.33E-09 5.55E-13
Y19 ENET_TXC PBIDIRHS_E33_33_NT_DR_V 0.3764 2.93E-09 6.88E-13
Y17 ENET_TX_CTL PBIDIRHS_E33_33_NT_DR_V 0.25907 2.12E-09 5.40E-13
V8 GPIO1_IO00 PBIDIRHS_E33_33_NT_DR_V 0.20458 1.35E-09 4.14E-13
R8 GPIO1_IO01 PBIDIRHS_E33_33_NT_DR_V 0.12697 8.83E-10 3.05E-13
AA8 GPIO1_IO02 PBIDIRHS_E33_33_NT_DR_V 0.24717 1.98E-09 4.64E-13
Y9 GPIO1_IO03 PBIDIRHS_E33_33_NT_DR_V 0.2701 2.01E-09 5.11E-13
AA7 GPIO1_IO04 PBIDIRHS_E33_33_NT_DR_V 0.28168 2.05E-09 4.85E-13
T8 GPIO1_IO05 PBIDIRHS_E33_33_NT_DR_V 0.18132 1.25E-09 3.55E-13
Y8 GPIO1_IO06 PBIDIRHS_E33_33_NT_DR_V 0.22537 1.73E-09 4.83E-13
U8 GPIO1_IO07 PBIDIRHS_E33_33_NT_DR_V 0.22716 1.58E-09 3.79E-13
V10 GPIO1_IO08 PBIDIRHS_E33_33_NT_DR_V 0.16439 1.29E-09 3.99E-13
AA9 GPIO1_IO09 PBIDIRHS_E33_33_NT_DR_V 0.3078 2.35E-09 5.54E-13
AA10 GPIO1_IO10 PBIDIRHS_E33_33_NT_DR_V 0.20705 1.76E-09 4.61E-13
Y11 GPIO1_IO11 PBIDIRHS_E33_33_NT_DR_V 0.27208 2.05E-09 5.26E-13
U10 GPIO1_IO12 PBIDIRHS_E33_33_NT_DR_V 0.14632 1.12E-09 3.48E-13
T10 GPIO1_IO13 PBIDIRHS_E33_33_NT_DR_V 0.15864 1.12E-09 3.45E-13
Y10 GPIO1_IO14 PBIDIRHS_E33_33_NT_DR_V 0.20307 1.64E-09 4.92E-13
AA11 GPIO1_IO15 PBIDIRHS_E33_33_NT_DR_V 0.31611 2.46E-09 6.06E-13
B7 I2C1_SCL PBIDIRHS_E33_33_NT_DR_V 0.18974 1.76E-09 5.44E-13
A7 I2C1_SDA PBIDIRHS_E33_33_NT_DR_V 0.20588 1.81E-09 5.43E-13
F10 I2C2_SCL PBIDIRHS_E33_33_NT_DR_V 0.042363 5.89E-10 2.43E-13
D8 I2C2_SDA PBIDIRHS_E33_33_NT_DR_V 0.10863 1.08E-09 3.72E-13
F8 I2C3_SCL PBIDIRHS_E33_33_NT_DR_V 0.0499 4.90E-10 2.77E-13
E8 I2C3_SDA PBIDIRHS_E33_33_NT_DR_V 0.088438 7.32E-10 3.47E-13
B8 I2C4_SCL PBIDIRHS_E33_33_NT_DR_V 0.16288 1.36E-09 4.84E-13
A8 I2C4_SDA PBIDIRHS_E33_33_NT_DR_V 0.18456 1.75E-09 5.11E-13
D18 JTAG_MOD PBIDIRHS_E33_33_NT_DR_V 0.4001 2.70E-09 7.16E-13
D21 JTAG_TCK PBIDIRHS_E33_33_NT_DR_V 0.31087 2.24E-09 6.30E-13
C21 JTAG_TDI PBIDIRHS_E33_33_NT_DR_V 0.33594 2.39E-09 6.74E-13
D20 JTAG_TDO PBIDIRHS_E33_33_NT_DR_V 0.36165 2.53E-09 6.48E-13
E18 JTAG_TMS PBIDIRHS_E33_33_NT_DR_V 0.30306 1.92E-09 5.32E-13
A13 MIPI_CSI_CLK_N DPHY_RX 0.26237 2.33E-09 4.36E-13
B13 MIPI_CSI_CLK_P DPHY_RX 0.24891 2.29E-09 4.34E-13
A11 MIPI_CSI_D0_N DPHY_RX 0.28063 2.36E-09 4.72E-13
B11 MIPI_CSI_D0_P DPHY_RX 0.28791 2.35E-09 4.69E-13
A12 MIPI_CSI_D1_N DPHY_RX 0.26791 2.34E-09 4.54E-13
B12 MIPI_CSI_D1_P DPHY_RX 0.27798 2.33E-09 4.50E-13
A14 MIPI_CSI_D2_N DPHY_RX 0.26816 2.42E-09 4.38E-13
B14 MIPI_CSI_D2_P DPHY_RX 0.25686 2.27E-09 4.50E-13
A15 MIPI_CSI_D3_N DPHY_RX 0.27241 2.27E-09 4.64E-13
B15 MIPI_CSI_D3_P DPHY_RX 0.26013 2.23E-09 4.63E-13
D12 MIPI_VREG_CAP NC 0.15542 1.25E-09 4.08E-13
J17 NAND_ALE PBIDIRHS_E33_33_NT_DR_H 0.26208 1.75E-09 5.21E-13
L21 NAND_CE0_B PBIDIRHS_E33_33_NT_DR_H 0.33506 2.35E-09 6.30E-13
H20 NAND_CE1_B PBIDIRHS_E33_33_NT_DR_H 0.36038 2.52E-09 7.05E-13
L16 NAND_CE2_B PBIDIRHS_E33_33_NT_DR_H 0.19015 1.27E-09 4.13E-13
L20 NAND_CE3_B PBIDIRHS_E33_33_NT_DR_H 0.20215 1.38E-09 4.43E-13
K20 NAND_CLE PBIDIRHS_E33_33_NT_DR_H 0.31347 2.16E-09 5.80E-13
M21 NAND_DATA00 PBIDIRHS_E33_33_NT_DR_H 0.21572 1.49E-09 4.86E-13
J20 NAND_DATA01 PBIDIRHS_E33_33_NT_DR_H 0.20196 1.37E-09 4.59E-13
M20 NAND_DATA02 PBIDIRHS_E33_33_NT_DR_H 0.21525 1.50E-09 4.62E-13
K21 NAND_DATA03 PBIDIRHS_E33_33_NT_DR_H 0.26148 1.88E-09 5.40E-13
L18 NAND_DATA04 PBIDIRHS_E33_33_NT_DR_H 0.27369 1.82E-09 5.27E-13
J18 NAND_DATA05 PBIDIRHS_E33_33_NT_DR_H 0.29229 2.01E-09 5.67E-13
N20 NAND_DATA06 PBIDIRHS_E33_33_NT_DR_H 0.20626 1.43E-09 4.33E-13
G20 NAND_DATA07 PBIDIRHS_E33_33_NT_DR_H 0.36005 2.56E-09 6.79E-13
H21 NAND_DQS PBIDIRHS_E33_33_NT_DR_H 0.28148 1.99E-09 5.84E-13
L17 NAND_READY_B PBIDIRHS_E33_33_NT_DR_H 0.17925 1.17E-09 4.20E-13
G21 NAND_RE_B PBIDIRHS_E33_33_NT_DR_H 0.39517 2.75E-09 7.06E-13
J16 NAND_WE_B PBIDIRHS_E33_33_NT_DR_H 0.18633 1.32E-09 4.48E-13
J21 NAND_WP_B PBIDIRHS_E33_33_NT_DR_H 0.23645 1.66E-09 5.17E-13
E14 ONOFF PINC_E33_33_NT_DR_H 0.16424 1.13E-09 4.24E-13
E16 PMIC_ON_REQ PBIDIR_E33_33_NT_DR_H 0.16409 1.04E-09 3.64E-13
A19 PMIC_STBY_REQ PBIDIR_E33_33_NT_DR_H 0.43946 3.06E-09 7.98E-13
A18 POR_B PINC_E33_33_NT_DR_H 0.32243 2.27E-09 6.13E-13
B18 RTC_RESET_B PINC_E33_33_NT_DR_H 0.25614 1.69E-09 5.34E-13
A20 RTC_XTALI NC 0.33765 2.31E-09 6.49E-13
B19 RTC_XTALO NC 0.30612 2.04E-09 5.79E-13
Y12 SAI2_MCLK PBIDIRHS_E33_33_NT_DR_V 0.19325 1.62E-09 4.53E-13
AA15 SAI2_RXC PBIDIRHS_E33_33_NT_DR_V 0.33495 2.58E-09 5.96E-13
AA14 SAI2_RXD0 PBIDIRHS_E33_33_NT_DR_V 0.31569 2.49E-09 5.55E-13
Y13 SAI2_RXFS PBIDIRHS_E33_33_NT_DR_V 0.20234 1.68E-09 4.83E-13
AA13 SAI2_TXC PBIDIRHS_E33_33_NT_DR_V 0.23704 1.99E-09 5.28E-13
Y14 SAI2_TXD0 PBIDIRHS_E33_33_NT_DR_V 0.29334 2.26E-09 5.60E-13
AA12 SAI2_TXFS PBIDIRHS_E33_33_NT_DR_V 0.28907 2.28E-09 4.99E-13
AA5 SAI3_MCLK PBIDIRHS_E33_33_NT_DR_V 0.24276 1.74E-09 4.77E-13
Y6 SAI3_RXC PBIDIRHS_E33_33_NT_DR_V 0.20365 1.38E-09 4.74E-13
AA6 SAI3_RXD PBIDIRHS_E33_33_NT_DR_V 0.23768 1.71E-09 4.55E-13
Y4 SAI3_RXFS PBIDIRHS_E33_33_NT_DR_V 0.21334 1.46E-09 5.09E-13
Y5 SAI3_TXC PBIDIRHS_E33_33_NT_DR_V 0.21435 1.43E-09 5.00E-13
AA4 SAI3_TXD PBIDIRHS_E33_33_NT_DR_V 0.23541 1.69E-09 5.07E-13
Y7 SAI3_TXFS PBIDIRHS_E33_33_NT_DR_V 0.2122 1.42E-09 4.70E-13
W11 SAI5_MCLK PBIDIRHS_E33_33_NT_DR_V 0.162 1.27E-09 3.70E-13
V14 SAI5_RXC PBIDIRHS_E33_33_NT_DR_V 0.3289 2.45E-09 6.69E-13
U12 SAI5_RXD0 PBIDIRHS_E33_33_NT_DR_V 0.1237 9.72E-10 3.38E-13
T14 SAI5_RXD1 PBIDIRHS_E33_33_NT_DR_V 0.28284 2.04E-09 5.76E-13
V12 SAI5_RXD2 PBIDIRHS_E33_33_NT_DR_V 0.17917 1.34E-09 4.37E-13
U14 SAI5_RXD3 PBIDIRHS_E33_33_NT_DR_V 0.29577 2.18E-09 6.25E-13
T12 SAI5_RXFS PBIDIRHS_E33_33_NT_DR_V 0.09729 8.19E-10 3.25E-13
R21 SD1_CLK PBIDIRHS_E33_33_NT_DR_V 0.18682 1.35E-09 4.84E-13
T21 SD1_CMD PBIDIRHS_E33_33_NT_DR_V 0.22967 2.05E-09 4.94E-13
N18 SD1_DATA0 PBIDIRHS_E33_33_NT_DR_V 0.17584 1.14E-09 4.24E-13
N17 SD1_DATA1 PBIDIRHS_E33_33_NT_DR_V 0.20657 1.36E-09 4.51E-13
N21 SD1_DATA2 PBIDIRHS_E33_33_NT_DR_V 0.20389 1.44E-09 4.74E-13
P20 SD1_DATA3 PBIDIRHS_E33_33_NT_DR_V 0.20405 1.41E-09 5.07E-13
P21 SD1_DATA4 PBIDIRHS_E33_33_NT_DR_V 0.20354 1.47E-09 4.86E-13
T20 SD1_DATA5 PBIDIRHS_E33_33_NT_DR_V 0.2197 1.95E-09 4.61E-13
R20 SD1_DATA6 PBIDIRHS_E33_33_NT_DR_V 0.24997 1.98E-09 5.34E-13
N16 SD1_DATA7 PBIDIRHS_E33_33_NT_DR_V 0.04496 3.37E-10 2.31E-13
R18 SD1_RESET_B PBIDIRHS_E33_33_NT_DR_V 0.15172 9.69E-10 3.75E-13
R17 SD1_STROBE PBIDIRHS_E33_33_NT_DR_V 0.10301 6.25E-10 2.87E-13
U20 SD2_CD_B PBIDIRHS_E33_33_NT_DR_V 0.30538 2.34E-09 5.60E-13
Y21 SD2_CLK PBIDIRHS_E33_33_NT_DR_V 0.32705 2.62E-09 6.79E-13
V21 SD2_CMD PBIDIRHS_E33_33_NT_DR_V 0.37916 2.92E-09 6.80E-13
AA20 SD2_DATA0 PBIDIRHS_E33_33_NT_DR_V 0.33361 2.71E-09 6.60E-13
U21 SD2_DATA1 PBIDIRHS_E33_33_NT_DR_V 0.35885 2.72E-09 6.40E-13
W20 SD2_DATA2 PBIDIRHS_E33_33_NT_DR_V 0.32183 2.59E-09 6.47E-13
V20 SD2_DATA3 PBIDIRHS_E33_33_NT_DR_V 0.3378 2.58E-09 6.18E-13
Y20 SD2_RESET_B PBIDIRHS_E33_33_NT_DR_V 0.3143 2.56E-09 6.32E-13
W21 SD2_WP PBIDIRHS_E33_33_NT_DR_V 0.32218 2.59E-09 6.44E-13
T6 SPDIF_EXT_CLK PBIDIRHS_E33_33_NT_DR_V 0.076372 5.04E-10 3.00E-13
U6 SPDIF_RX PBIDIRHS_E33_33_NT_DR_V 0.15092 9.36E-10 3.78E-13
V6 SPDIF_TX PBIDIRHS_E33_33_NT_DR_V 0.17805 1.18E-09 4.22E-13
D16 TSENSOR_RES_EXT NC 0.32227 2.13E-09 5.47E-13
A9 UART1_RXD PBIDIRHS_E33_33_NT_DR_V 0.19859 1.75E-09 5.23E-13
E10 UART1_TXD PBIDIRHS_E33_33_NT_DR_V 0.07113 7.72E-10 3.06E-13
B9 UART2_RXD PBIDIRHS_E33_33_NT_DR_V 0.17239 1.49E-09 4.98E-13
C11 UART2_TXD PBIDIRHS_E33_33_NT_DR_V 0.11693 1.16E-09 4.28E-13
B10 UART3_RXD PBIDIRHS_E33_33_NT_DR_V 0.17308 1.41E-09 4.83E-13
E12 UART3_TXD PBIDIRHS_E33_33_NT_DR_V 0.099087 9.18E-10 3.83E-13
A10 UART4_RXD PBIDIRHS_E33_33_NT_DR_V 0.19623 1.59E-09 5.29E-13
D10 UART4_TXD PBIDIRHS_E33_33_NT_DR_V 0.10519 1.06E-09 3.79E-13
A17 USB1_DN USB2_HS_IBIS 0.25063 2.11E-09 4.76E-13
B17 USB1_DP USB2_HS_IBIS 0.25274 2.10E-09 4.59E-13
D14 USB1_ID NC 0.19059 1.43E-09 4.46E-13
B16 USB1_TXRTUNE NC 0.21826 1.61E-09 5.08E-13
A16 USB1_VBUS NC 0.23355 1.89E-09 5.20E-13
A1 VSS GND
A21 VSS GND
AA1 VSS GND
AA21 VSS GND
B20 VSS GND
C4 VSS GND
C6 VSS GND
C8 VSS GND
C10 VSS GND
C12 VSS GND
C14 VSS GND
C16 VSS GND
C18 VSS GND
E3 VSS GND
E19 VSS GND
G3 VSS GND
G19 VSS GND
H8 VSS GND
H10 VSS GND
H12 VSS GND
H14 VSS GND
J3 VSS GND
J8 VSS GND
J14 VSS GND
J19 VSS GND
K11 VSS GND
L3 VSS GND
L8 VSS GND
L14 VSS GND
L19 VSS GND
M11 VSS GND
N3 VSS GND
N8 VSS GND
N14 VSS GND
N19 VSS GND
P8 VSS GND
P10 VSS GND
P12 VSS GND
P14 VSS GND
R3 VSS GND
R19 VSS GND
U3 VSS GND
U19 VSS GND
W4 VSS GND
W6 VSS GND
W8 VSS GND
W10 VSS GND
W12 VSS GND
W14 VSS GND
W16 VSS GND
W18 VSS GND
[Diff_pin] inv_pin vdiff tdelay_typ tdelay_min tdelay_max
G5 G4 0.140V 0ns NA NA
J4 J5 0.140V 0ns NA NA
T1 T2 0.140V 0ns NA NA
Y2 AA2 0.140V 0ns NA NA
B1 C2 0.140V 0ns NA NA
G2 F1 0.140V 0ns NA NA
B13 A13 NA NA NA NA
B11 A11 NA NA NA NA
B12 A12 NA NA NA NA
B14 A14 NA NA NA NA
B15 A15 NA NA NA NA
B17 A17 150.000mV 0ns NA NA
|END COMPONENT
[Model Selector] DQ_DQS
mal4drv27_d3l_28   DDR3L mal4drv27 cell  Z0=28-Ohm Driver
mal4drv27_d3l_34   DDR3L mal4drv27 cell  Z0=34-Ohm Driver
mal4drv27_d3l_40   DDR3L mal4drv27 cell  Z0=40-Ohm Driver
mal4drv27_d3l_53   DDR3L mal4drv27 cell  Z0=53-Ohm Driver
mal4drv27_d3l_60   DDR3L mal4drv27 cell  Z0=60-Ohm Driver
mal4drv27_d3l_odt120   DDR3L mal4drv27 cell 120-Ohm ODT Receiver
mal4drv27_d3l_odt60   DDR3L mal4drv27 cell 60-Ohm ODT Receiver
mal4drv27_d4_28   DDR4 mal4drv27 cell  Z0=28-Ohm Driver
mal4drv27_d4_34   DDR4 mal4drv27 cell  Z0=34-Ohm Driver
mal4drv27_d4_40   DDR4 mal4drv27 cell  Z0=40-Ohm Driver
mal4drv27_d4_53   DDR4 mal4drv27 cell  Z0=53-Ohm Driver
mal4drv27_d4_60   DDR4 mal4drv27 cell  Z0=60-Ohm Driver
mal4drv27_d4_odt120   DDR4 mal4drv27 cell 120-Ohm ODT Receiver
mal4drv27_d4_odt240   DDR4 mal4drv27 cell 240-Ohm ODT Receiver
mal4drv27_d4_odt48   DDR4 mal4drv27 cell 48-Ohm ODT Receiver
mal4drv27_d4_odt60   DDR4 mal4drv27 cell 60-Ohm ODT Receiver
mal4drv27_d4_odt80   DDR4 mal4drv27 cell 80-Ohm ODT Receiver
mal4drv27_dl4_28   LPDDR4 mal4drv27 cell  Z0=28-Ohm Driver
mal4drv27_dl4_34   LPDDR4 mal4drv27 cell  Z0=34-Ohm Driver
mal4drv27_dl4_40   LPDDR4 mal4drv27 cell  Z0=40-Ohm Driver
mal4drv27_dl4_53   LPDDR4 mal4drv27 cell  Z0=53-Ohm Driver
mal4drv27_dl4_60   LPDDR4 mal4drv27 cell  Z0=60-Ohm Driver
mal4drv27_dl4_odt48   LPDDR4 mal4drv27 cell 48-Ohm ODT Receiver
mal4drv27_dl4_odt60   LPDDR4 mal4drv27 cell 60-Ohm ODT Receiver
[Model Selector] CA_CK
mal4drv20_d3l_20   DDR3L mal4drv20 cell  Z0=20-Ohm Driver
mal4drv20_d3l_24   DDR3L mal4drv20 cell  Z0=24-Ohm Driver
mal4drv20_d3l_30   DDR3L mal4drv20 cell  Z0=30-Ohm Driver
mal4drv20_d3l_40   DDR3L mal4drv20 cell  Z0=40-Ohm Driver
mal4drv20_d3l_60   DDR3L mal4drv20 cell  Z0=60-Ohm Driver
mal4drv20_d4_20   DDR4 mal4drv20 cell  Z0=20-Ohm Driver
mal4drv20_d4_24   DDR4 mal4drv20 cell  Z0=24-Ohm Driver
mal4drv20_d4_30   DDR4 mal4drv20 cell  Z0=30-Ohm Driver
mal4drv20_d4_40   DDR4 mal4drv20 cell  Z0=40-Ohm Driver
mal4drv20_d4_60   DDR4 mal4drv20 cell  Z0=60-Ohm Driver
mal4drv20_dl4_20   LPDDR4 mal4drv20 cell  Z0=20-Ohm Driver
mal4drv20_dl4_24   LPDDR4 mal4drv20 cell  Z0=24-Ohm Driver
mal4drv20_dl4_30   LPDDR4 mal4drv20 cell  Z0=30-Ohm Driver
mal4drv20_dl4_40   LPDDR4 mal4drv20 cell  Z0=40-Ohm Driver
mal4drv20_dl4_60   LPDDR4 mal4drv20 cell  Z0=60-Ohm Driver
[Model Selector] USB2_HS_IBIS
USB2_HSRX   USB2 HS RX model
USB2_HSTX_00_0_01_0011_11   USB2 HS TX model: AMP_PULSE_RISE_VREF_XV=00_0_01_0011_11
[Model Selector] PBIDIR_E33_33_NT_DR_H
| Model Description
M0_PBIDIR_E33_DR_0_1P80V   - 2mA drive strength, fast output slew: - without weak pull
M1_PBIDIR_E33_DR_0_1P80V   - 2mA drive strength, fast output slew: - with weak pulldown
M2_PBIDIR_E33_DR_0_1P80V   - 2mA drive strength, fast output slew: - with weak pullup
M3_PBIDIR_E33_DR_0_1P80V   - 2mA drive strength, slow output slew: - without weak pull
M4_PBIDIR_E33_DR_0_1P80V   - 2mA drive strength, slow output slew: - with weak pulldown
M5_PBIDIR_E33_DR_0_1P80V   - 2mA drive strength, slow output slew: - with weak pullup
M6_PBIDIR_E33_DR_0_1P80V   - 4mA drive strength, fast output slew: - without weak pull
M7_PBIDIR_E33_DR_0_1P80V   - 4mA drive strength, fast output slew: - with weak pulldown
M8_PBIDIR_E33_DR_0_1P80V   - 4mA drive strength, fast output slew: - with weak pullup
M9_PBIDIR_E33_DR_0_1P80V   - 4mA drive strength, slow output slew: - without weak pull
M10_PBIDIR_E33_DR_1P80V   - 4mA drive strength, slow output slew: - with weak pulldown
M11_PBIDIR_E33_DR_1P80V   - 4mA drive strength, slow output slew: - with weak pullup
M12_PBIDIR_E33_DR_1P80V   - 8mA drive strength, fast output slew: - without weak pull
M13_PBIDIR_E33_DR_1P80V   - 8mA drive strength, fast output slew: - with weak pulldown
M14_PBIDIR_E33_DR_1P80V   - 8mA drive strength, fast output slew: - with weak pullup
M15_PBIDIR_E33_DR_1P80V   - 8mA drive strength, slow output slew: - without weak pull
M16_PBIDIR_E33_DR_1P80V   - 8mA drive strength, slow output slew: - with weak pulldown
M17_PBIDIR_E33_DR_1P80V   - 8mA drive strength, slow output slew: - with weak pullup
M18_PBIDIR_E33_DR_1P80V   - 12mA drive strength, fast output slew: - without weak pull
M19_PBIDIR_E33_DR_1P80V   - 12mA drive strength, fast output slew: - with weak pulldown
M20_PBIDIR_E33_DR_1P80V   - 12mA drive strength, fast output slew: - with weak pullup
M21_PBIDIR_E33_DR_1P80V   - 12mA drive strength, slow output slew: - without weak pull
M22_PBIDIR_E33_DR_1P80V   - 12mA drive strength, slow output slew: - with weak pulldown
M23_PBIDIR_E33_DR_1P80V   - 12mA drive strength, slow output slew: - with weak pullup
M0_PBIDIR_E33_DR_0_3P30V   - 2mA drive strength, fast output slew: - without weak pull
M1_PBIDIR_E33_DR_0_3P30V   - 2mA drive strength, fast output slew: - with weak pulldown
M2_PBIDIR_E33_DR_0_3P30V   - 2mA drive strength, fast output slew: - with weak pullup
M3_PBIDIR_E33_DR_0_3P30V   - 2mA drive strength, slow output slew: - without weak pull
M4_PBIDIR_E33_DR_0_3P30V   - 2mA drive strength, slow output slew: - with weak pulldown
M5_PBIDIR_E33_DR_0_3P30V   - 2mA drive strength, slow output slew: - with weak pullup
M6_PBIDIR_E33_DR_0_3P30V   - 4mA drive strength, fast output slew: - without weak pull
M7_PBIDIR_E33_DR_0_3P30V   - 4mA drive strength, fast output slew: - with weak pulldown
M8_PBIDIR_E33_DR_0_3P30V   - 4mA drive strength, fast output slew: - with weak pullup
M9_PBIDIR_E33_DR_0_3P30V   - 4mA drive strength, slow output slew: - without weak pull
M10_PBIDIR_E33_DR_3P30V   - 4mA drive strength, slow output slew: - with weak pulldown
M11_PBIDIR_E33_DR_3P30V   - 4mA drive strength, slow output slew: - with weak pullup
M12_PBIDIR_E33_DR_3P30V   - 8mA drive strength, fast output slew: - without weak pull
M13_PBIDIR_E33_DR_3P30V   - 8mA drive strength, fast output slew: - with weak pulldown
M14_PBIDIR_E33_DR_3P30V   - 8mA drive strength, fast output slew: - with weak pullup
M15_PBIDIR_E33_DR_3P30V   - 8mA drive strength, slow output slew: - without weak pull
M16_PBIDIR_E33_DR_3P30V   - 8mA drive strength, slow output slew: - with weak pulldown
M17_PBIDIR_E33_DR_3P30V   - 8mA drive strength, slow output slew: - with weak pullup
M18_PBIDIR_E33_DR_3P30V   - 12mA drive strength, fast output slew: - without weak pull
M19_PBIDIR_E33_DR_3P30V   - 12mA drive strength, fast output slew: - with weak pulldown
M20_PBIDIR_E33_DR_3P30V   - 12mA drive strength, fast output slew: - with weak pullup
M21_PBIDIR_E33_DR_3P30V   - 12mA drive strength, slow output slew: - without weak pull
M22_PBIDIR_E33_DR_3P30V   - 12mA drive strength, slow output slew: - with weak pulldown
M23_PBIDIR_E33_DR_3P30V   - 12mA drive strength, slow output slew: - with weak pullup
[Model Selector] PBIDIRHS_E33_33_NT_DR_H
| Model Description
M0_PBIDIR_HS_02_F_1P80V_H   - 2mA drive strength, fast output slew: - without weak pull
M1_PBIDIR_HS_02_F_1P80V_H   - 2mA drive strength, fast output slew: - with weak pulldown
M2_PBIDIR_HS_02_F_1P80V_H   - 2mA drive strength, fast output slew: - with weak pullup
M3_PBIDIR_HS_02_S_1P80V_H   - 2mA drive strength, slow output slew: - without weak pull
M4_PBIDIR_HS_02_S_1P80V_H   - 2mA drive strength, slow output slew: - with weak pulldown
M5_PBIDIR_HS_02_S_1P80V_H   - 2mA drive strength, slow output slew: - with weak pullup
M6_PBIDIR_HS_04_F_1P80V_H   - 4mA drive strength, fast output slew: - without weak pull
M7_PBIDIR_HS_04_F_1P80V_H   - 4mA drive strength, fast output slew: - with weak pulldown
M8_PBIDIR_HS_04_F_1P80V_H   - 4mA drive strength, fast output slew: - with weak pullup
M9_PBIDIR_HS_04_S_1P80V_H   - 4mA drive strength, slow output slew: - without weak pull
M10_PBIDIR_HS_04_S_1P80V_H   - 4mA drive strength, slow output slew: - with weak pulldown
M11_PBIDIR_HS_04_S_1P80V_H   - 4mA drive strength, slow output slew: - with weak pullup
M12_PBIDIR_HS_08_F_1P80V_H   - 8mA drive strength, fast output slew: - without weak pull
M13_PBIDIR_HS_08_F_1P80V_H   - 8mA drive strength, fast output slew: - with weak pulldown
M14_PBIDIR_HS_08_F_1P80V_H   - 8mA drive strength, fast output slew: - with weak pullup
M15_PBIDIR_HS_08_S_1P80V_H   - 8mA drive strength, slow output slew: - without weak pull
M16_PBIDIR_HS_08_S_1P80V_H   - 8mA drive strength, slow output slew: - with weak pulldown
M17_PBIDIR_HS_08_S_1P80V_H   - 8mA drive strength, slow output slew: - with weak pullup
M18_PBIDIR_HS_12_F_1P80V_H   - 12mA drive strength, fast output slew: - without weak pull
M19_PBIDIR_HS_12_F_1P80V_H   - 12mA drive strength, fast output slew: - with weak pulldown
M20_PBIDIR_HS_12_F_1P80V_H   - 12mA drive strength, fast output slew: - with weak pullup
M21_PBIDIR_HS_12_S_1P80V_H   - 12mA drive strength, slow output slew: - without weak pull
M22_PBIDIR_HS_12_S_1P80V_H   - 12mA drive strength, slow output slew: - with weak pulldown
M23_PBIDIR_HS_12_S_1P80V_H   - 12mA drive strength, slow output slew: - with weak pullup
M0_PBIDIR_HS_02_F_3P30V_H   - 2mA drive strength, fast output slew: - without weak pull
M1_PBIDIR_HS_02_F_3P30V_H   - 2mA drive strength, fast output slew: - with weak pulldown
M2_PBIDIR_HS_02_F_3P30V_H   - 2mA drive strength, fast output slew: - with weak pullup
M3_PBIDIR_HS_02_S_3P30V_H   - 2mA drive strength, slow output slew: - without weak pull
M4_PBIDIR_HS_02_S_3P30V_H   - 2mA drive strength, slow output slew: - with weak pulldown
M5_PBIDIR_HS_02_S_3P30V_H   - 2mA drive strength, slow output slew: - with weak pullup
M6_PBIDIR_HS_04_F_3P30V_H   - 4mA drive strength, fast output slew: - without weak pull
M7_PBIDIR_HS_04_F_3P30V_H   - 4mA drive strength, fast output slew: - with weak pulldown
M8_PBIDIR_HS_04_F_3P30V_H   - 4mA drive strength, fast output slew: - with weak pullup
M9_PBIDIR_HS_04_S_3P30V_H   - 4mA drive strength, slow output slew: - without weak pull
M10_PBIDIR_HS_04_S_3P30V_H   - 4mA drive strength, slow output slew: - with weak pulldown
M11_PBIDIR_HS_04_S_3P30V_H   - 4mA drive strength, slow output slew: - with weak pullup
M12_PBIDIR_HS_08_F_3P30V_H   - 8mA drive strength, fast output slew: - without weak pull
M13_PBIDIR_HS_08_F_3P30V_H   - 8mA drive strength, fast output slew: - with weak pulldown
M14_PBIDIR_HS_08_F_3P30V_H   - 8mA drive strength, fast output slew: - with weak pullup
M15_PBIDIR_HS_08_S_3P30V_H   - 8mA drive strength, slow output slew: - without weak pull
M16_PBIDIR_HS_08_S_3P30V_H   - 8mA drive strength, slow output slew: - with weak pulldown
M17_PBIDIR_HS_08_S_3P30V_H   - 8mA drive strength, slow output slew: - with weak pullup
M18_PBIDIR_HS_12_F_3P30V_H   - 12mA drive strength, fast output slew: - without weak pull
M19_PBIDIR_HS_12_F_3P30V_H   - 12mA drive strength, fast output slew: - with weak pulldown
M20_PBIDIR_HS_12_F_3P30V_H   - 12mA drive strength, fast output slew: - with weak pullup
M21_PBIDIR_HS_12_S_3P30V_H   - 12mA drive strength, slow output slew: - without weak pull
M22_PBIDIR_HS_12_S_3P30V_H   - 12mA drive strength, slow output slew: - with weak pulldown
M23_PBIDIR_HS_12_S_3P30V_H   - 12mA drive strength, slow output slew: - with weak pullup
[Model Selector] PBIDIRHS_E33_33_NT_DR_V
| Model Description
M0_PBIDIR_HS_02_F_1P80V_V   - 2mA drive strength, fast output slew: - without weak pull
M1_PBIDIR_HS_02_F_1P80V_V   - 2mA drive strength, fast output slew: - with weak pulldown
M2_PBIDIR_HS_02_F_1P80V_V   - 2mA drive strength, fast output slew: - with weak pullup
M3_PBIDIR_HS_02_S_1P80V_V   - 2mA drive strength, slow output slew: - without weak pull
M4_PBIDIR_HS_02_S_1P80V_V   - 2mA drive strength, slow output slew: - with weak pulldown
M5_PBIDIR_HS_02_S_1P80V_V   - 2mA drive strength, slow output slew: - with weak pullup
M6_PBIDIR_HS_04_F_1P80V_V   - 4mA drive strength, fast output slew: - without weak pull
M7_PBIDIR_HS_04_F_1P80V_V   - 4mA drive strength, fast output slew: - with weak pulldown
M8_PBIDIR_HS_04_F_1P80V_V   - 4mA drive strength, fast output slew: - with weak pullup
M9_PBIDIR_HS_04_S_1P80V_V   - 4mA drive strength, slow output slew: - without weak pull
M10_PBIDIR_HS_04_S_1P80V_V   - 4mA drive strength, slow output slew: - with weak pulldown
M11_PBIDIR_HS_04_S_1P80V_V   - 4mA drive strength, slow output slew: - with weak pullup
M12_PBIDIR_HS_08_F_1P80V_V   - 8mA drive strength, fast output slew: - without weak pull
M13_PBIDIR_HS_08_F_1P80V_V   - 8mA drive strength, fast output slew: - with weak pulldown
M14_PBIDIR_HS_08_F_1P80V_V   - 8mA drive strength, fast output slew: - with weak pullup
M15_PBIDIR_HS_08_S_1P80V_V   - 8mA drive strength, slow output slew: - without weak pull
M16_PBIDIR_HS_08_S_1P80V_V   - 8mA drive strength, slow output slew: - with weak pulldown
M17_PBIDIR_HS_08_S_1P80V_V   - 8mA drive strength, slow output slew: - with weak pullup
M18_PBIDIR_HS_12_F_1P80V_V   - 12mA drive strength, fast output slew: - without weak pull
M19_PBIDIR_HS_12_F_1P80V_V   - 12mA drive strength, fast output slew: - with weak pulldown
M20_PBIDIR_HS_12_F_1P80V_V   - 12mA drive strength, fast output slew: - with weak pullup
M21_PBIDIR_HS_12_S_1P80V_V   - 12mA drive strength, slow output slew: - without weak pull
M22_PBIDIR_HS_12_S_1P80V_V   - 12mA drive strength, slow output slew: - with weak pulldown
M23_PBIDIR_HS_12_S_1P80V_V   - 12mA drive strength, slow output slew: - with weak pullup
M0_PBIDIR_HS_02_F_3P30V_V   - 2mA drive strength, fast output slew: - without weak pull
M1_PBIDIR_HS_02_F_3P30V_V   - 2mA drive strength, fast output slew: - with weak pulldown
M2_PBIDIR_HS_02_F_3P30V_V   - 2mA drive strength, fast output slew: - with weak pullup
M3_PBIDIR_HS_02_S_3P30V_V   - 2mA drive strength, slow output slew: - without weak pull
M4_PBIDIR_HS_02_S_3P30V_V   - 2mA drive strength, slow output slew: - with weak pulldown
M5_PBIDIR_HS_02_S_3P30V_V   - 2mA drive strength, slow output slew: - with weak pullup
M6_PBIDIR_HS_04_F_3P30V_V   - 4mA drive strength, fast output slew: - without weak pull
M7_PBIDIR_HS_04_F_3P30V_V   - 4mA drive strength, fast output slew: - with weak pulldown
M8_PBIDIR_HS_04_F_3P30V_V   - 4mA drive strength, fast output slew: - with weak pullup
M9_PBIDIR_HS_04_S_3P30V_V   - 4mA drive strength, slow output slew: - without weak pull
M10_PBIDIR_HS_04_S_3P30V_V   - 4mA drive strength, slow output slew: - with weak pulldown
M11_PBIDIR_HS_04_S_3P30V_V   - 4mA drive strength, slow output slew: - with weak pullup
M12_PBIDIR_HS_08_F_3P30V_V   - 8mA drive strength, fast output slew: - without weak pull
M13_PBIDIR_HS_08_F_3P30V_V   - 8mA drive strength, fast output slew: - with weak pulldown
M14_PBIDIR_HS_08_F_3P30V_V   - 8mA drive strength, fast output slew: - with weak pullup
M15_PBIDIR_HS_08_S_3P30V_V   - 8mA drive strength, slow output slew: - without weak pull
M16_PBIDIR_HS_08_S_3P30V_V   - 8mA drive strength, slow output slew: - with weak pulldown
M17_PBIDIR_HS_08_S_3P30V_V   - 8mA drive strength, slow output slew: - with weak pullup
M18_PBIDIR_HS_12_F_3P30V_V   - 12mA drive strength, fast output slew: - without weak pull
M19_PBIDIR_HS_12_F_3P30V_V   - 12mA drive strength, fast output slew: - with weak pulldown
M20_PBIDIR_HS_12_F_3P30V_V   - 12mA drive strength, fast output slew: - with weak pullup
M21_PBIDIR_HS_12_S_3P30V_V   - 12mA drive strength, slow output slew: - without weak pull
M22_PBIDIR_HS_12_S_3P30V_V   - 12mA drive strength, slow output slew: - with weak pulldown
M23_PBIDIR_HS_12_S_3P30V_V   - 12mA drive strength, slow output slew: - with weak pullup
| Submodel
[Submodel]  M1_PBIDIR_E33_DR_0_1P80V_T
Submodel_type Dynamic_clamp
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| Submodel
[Submodel]  M2_PBIDIR_E33_DR_0_1P80V_T
Submodel_type Dynamic_clamp
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| Submodel
[Submodel]  M4_PBIDIR_E33_DR_0_1P80V_T
Submodel_type Dynamic_clamp
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| Submodel
[Submodel]  M5_PBIDIR_E33_DR_0_1P80V_T
Submodel_type Dynamic_clamp
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| Submodel
[Submodel]  M7_PBIDIR_E33_DR_0_1P80V_T
Submodel_type Dynamic_clamp
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| Submodel
[Submodel]  M8_PBIDIR_E33_DR_0_1P80V_T
Submodel_type Dynamic_clamp
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| Submodel
[Submodel]  M10_PBIDIR_E33_DR_1P80V_T
Submodel_type Dynamic_clamp
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| Submodel
[Submodel]  M11_PBIDIR_E33_DR_1P80V_T
Submodel_type Dynamic_clamp
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| Submodel
[Submodel]  M13_PBIDIR_E33_DR_1P80V_T
Submodel_type Dynamic_clamp
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| Submodel
[Submodel]  M14_PBIDIR_E33_DR_1P80V_T
Submodel_type Dynamic_clamp
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| Submodel
[Submodel]  M16_PBIDIR_E33_DR_1P80V_T
Submodel_type Dynamic_clamp
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| Submodel
[Submodel]  M17_PBIDIR_E33_DR_1P80V_T
Submodel_type Dynamic_clamp
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| Submodel
[Submodel]  M19_PBIDIR_E33_DR_1P80V_T
Submodel_type Dynamic_clamp
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| Submodel
[Submodel]  M20_PBIDIR_E33_DR_1P80V_T
Submodel_type Dynamic_clamp
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| Submodel
[Submodel]  M22_PBIDIR_E33_DR_1P80V_T
Submodel_type Dynamic_clamp
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| Submodel
[Submodel]  M23_PBIDIR_E33_DR_1P80V_T
Submodel_type Dynamic_clamp
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| Submodel
[Submodel]  M1_PBIDIR_E33_DR_0_3P30V_T
Submodel_type Dynamic_clamp
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| Submodel
[Submodel]  M4_PBIDIR_E33_DR_0_3P30V_T
Submodel_type Dynamic_clamp
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| Submodel
[Submodel]  M7_PBIDIR_E33_DR_0_3P30V_T
Submodel_type Dynamic_clamp
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| Submodel
[Submodel]  M10_PBIDIR_E33_DR_3P30V_T
Submodel_type Dynamic_clamp
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| Submodel
[Submodel]  M13_PBIDIR_E33_DR_3P30V_T
Submodel_type Dynamic_clamp
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| Submodel
[Submodel]  M16_PBIDIR_E33_DR_3P30V_T
Submodel_type Dynamic_clamp
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| Submodel
[Submodel]  M19_PBIDIR_E33_DR_3P30V_T
Submodel_type Dynamic_clamp
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| Submodel
[Submodel]  M22_PBIDIR_E33_DR_3P30V_T
Submodel_type Dynamic_clamp
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| Models and submodels in the file (284): mal4drv27_d3l_28 (I/O), mal4drv27_d3l_34 (I/O), mal4drv27_d3l_40 (I/O), mal4drv27_d3l_53 (I/O), mal4drv27_d3l_60 (I/O), mal4drv27_d3l_odt120 (Input), mal4drv27_d3l_odt60 (Input), mal4drv27_d4_28 (I/O), mal4drv27_d4_34 (I/O), mal4drv27_d4_40 (I/O), mal4drv27_d4_53 (I/O), mal4drv27_d4_60 (I/O), mal4drv27_d4_odt120 (Input), mal4drv27_d4_odt240 (Input), mal4drv27_d4_odt48 (Input), mal4drv27_d4_odt60 (Input), mal4drv27_d4_odt80 (Input), mal4drv27_dl4_28 (I/O), mal4drv27_dl4_34 (I/O), mal4drv27_dl4_40 (I/O), mal4drv27_dl4_53 (I/O), mal4drv27_dl4_60 (I/O), mal4drv27_dl4_odt48 (Input), mal4drv27_dl4_odt60 (Input), mal4drv20_d3l_20 (I/O), mal4drv20_d3l_24 (I/O), mal4drv20_d3l_30 (I/O), mal4drv20_d3l_40 (I/O), mal4drv20_d3l_60 (I/O), mal4drv20_d4_20 (I/O), mal4drv20_d4_24 (I/O), mal4drv20_d4_30 (I/O), mal4drv20_d4_40 (I/O), mal4drv20_d4_60 (I/O), mal4drv20_dl4_20 (I/O), mal4drv20_dl4_24 (I/O), mal4drv20_dl4_30 (I/O), mal4drv20_dl4_40 (I/O), mal4drv20_dl4_60 (I/O), DPHY_TX (Output), DPHY_RX (Input), USB2_HSRX (Input), USB2_HSTX_00_0_01_0011_11 (Output), PINC_E33_33_NT_DR_H (Input), M0_PBIDIR_E33_DR_0_1P80V (I/O), M1_PBIDIR_E33_DR_0_1P80V (I/O), M1_PBIDIR_E33_DR_0_1P80V_T (Dynamic_clamp), M2_PBIDIR_E33_DR_0_1P80V (I/O), M2_PBIDIR_E33_DR_0_1P80V_T (Dynamic_clamp), M3_PBIDIR_E33_DR_0_1P80V (I/O), M4_PBIDIR_E33_DR_0_1P80V (I/O), M4_PBIDIR_E33_DR_0_1P80V_T (Dynamic_clamp), M5_PBIDIR_E33_DR_0_1P80V (I/O), M5_PBIDIR_E33_DR_0_1P80V_T (Dynamic_clamp), M6_PBIDIR_E33_DR_0_1P80V (I/O), M7_PBIDIR_E33_DR_0_1P80V (I/O), M7_PBIDIR_E33_DR_0_1P80V_T (Dynamic_clamp), M8_PBIDIR_E33_DR_0_1P80V (I/O), M8_PBIDIR_E33_DR_0_1P80V_T (Dynamic_clamp), M9_PBIDIR_E33_DR_0_1P80V (I/O), M10_PBIDIR_E33_DR_1P80V (I/O), M10_PBIDIR_E33_DR_1P80V_T (Dynamic_clamp), M11_PBIDIR_E33_DR_1P80V (I/O), M11_PBIDIR_E33_DR_1P80V_T (Dynamic_clamp), M12_PBIDIR_E33_DR_1P80V (I/O), M13_PBIDIR_E33_DR_1P80V (I/O), M13_PBIDIR_E33_DR_1P80V_T (Dynamic_clamp), M14_PBIDIR_E33_DR_1P80V (I/O), M14_PBIDIR_E33_DR_1P80V_T (Dynamic_clamp), M15_PBIDIR_E33_DR_1P80V (I/O), M16_PBIDIR_E33_DR_1P80V (I/O), M16_PBIDIR_E33_DR_1P80V_T (Dynamic_clamp), M17_PBIDIR_E33_DR_1P80V (I/O), M17_PBIDIR_E33_DR_1P80V_T (Dynamic_clamp), M18_PBIDIR_E33_DR_1P80V (I/O), M19_PBIDIR_E33_DR_1P80V (I/O), M19_PBIDIR_E33_DR_1P80V_T (Dynamic_clamp), M20_PBIDIR_E33_DR_1P80V (I/O), M20_PBIDIR_E33_DR_1P80V_T (Dynamic_clamp), M21_PBIDIR_E33_DR_1P80V (I/O)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
